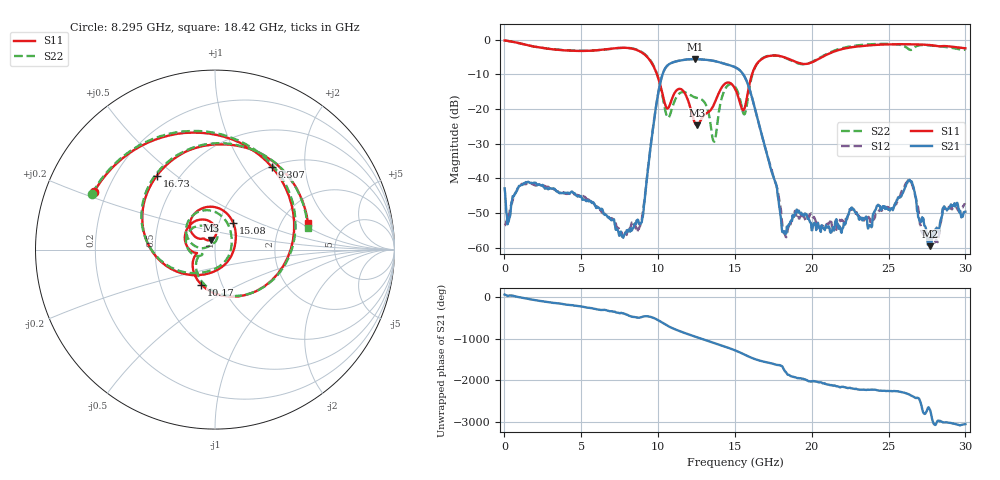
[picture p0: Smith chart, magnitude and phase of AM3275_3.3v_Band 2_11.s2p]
!Keysight Technologies,N5245B,MY58422270,A.16.20.02
!Date: Thursday, March 27, 2025 01:54:47
!Correction: S11(C  2-Port  )
!S21(C  2-Port  )
!S12(C  2-Port  )
!S22(C  2-Port  )
!S2P File: Measurements: S11, S21, S12, S22:
# Hz S  dB  R 50
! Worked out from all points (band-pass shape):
!   801 points, 10 MHz to 30 GHz, reference 50 ohm
!   highest |S21| = -5.59 dB at 12.38 GHz (marker M1); lowest = -59.6 dB at 27.71 GHz (marker M2)
!   |S21| within 3 dB of the highest: 10.42 GHz to 15.26 GHz (4.837 GHz wide, 37.7 % of centre)
!   lowest |S11| = -24.6 dB at 12.53 GHz (marker M3), VSWR 1.12, Z = 47.5 + j5.16 ohm
!   |S11| at or under -10 dB: 9.927 GHz to 16.11 GHz (6.183 GHz wide, 47.5 % of centre)
!   |S22| runs from -29.4 to -0.2 dB; largest |S21 - S12| = 0.0088
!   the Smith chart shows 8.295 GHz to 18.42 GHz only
!   S11 on the Smith chart (normalised r, x): 8.295 GHz: 0.15, +0.22; 9.307 GHz: 1.01, +1.36; 10.17 GHz: 0.80, -0.33; 15.08 GHz: 1.16, +0.36; 16.73 GHz: 0.38, +0.43; 18.42 GHz: 2.78, +1.17
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1e7  -0.20 -5.3  -42.87 49.9  -53.58 -84.8  -0.20 -6.2
9.097e8  -0.92 -86.4  -42.54 -10.0  -42.63 -6.4  -0.96 -86.3
2.071812e9  -2.08 -170.8  -41.58 -87.7  -42.06 -87.3  -2.08 -170.5
5.033325e9  -3.23 26.2  -45.60 123.8  -44.97 118.4  -3.18 25.1
6.832725e9  -2.63 -91.7  -51.58 12.4  -51.35 19.2  -2.68 -92.4
8.294738e9  -2.54 154.6  -55.01 -115.7  -52.72 -117.3  -2.48 155.5
9.3069e9  -5.05 55.6  -38.67 -107.2  -38.55 -105.5  -4.88 56.2
1.001916e10  -11.22 -72.6  -15.16 155.1  -15.13 154.9  -11.10 -68.5
1.016911e10  -13.54 -111.0  -11.92 122.0  -11.89 121.8  -13.69 -105.3
1.136871e10  -14.18 137.1  -6.04 -97.9  -6.03 -98.0  -15.55 165.9
1.238088e10  -23.88 96.9  -5.59 129.7  -5.58 129.7  -16.59 116.1
1.253082e10  -24.65 112.6  -5.60 111.2  -5.59 111.2  -16.78 112.7
1.346801e10  -20.01 143.2  -5.98 -2.3  -5.97 -2.5  -26.18 83.0
1.5005e10  -14.13 63.8  -7.92 159.1  -7.90 159.0  -13.54 90.2
1.507998e10  -14.85 56.1  -8.08 147.8  -8.06 147.8  -14.05 83.1
1.672942e10  -5.62 128.2  -27.11 -97.3  -27.19 -97.5  -5.53 129.9
1.841636e10  -5.37 16.1  -54.40 -55.8  -55.48 -76.4  -5.51 13.3
2.002832e10  -6.48 -124.8  -55.01 136.9  -50.77 145.5  -6.37 -128.1
2.253999e10  -2.20 102.7  -48.84 -24.1  -48.80 -20.3  -1.90 104.1
2.501416e10  -1.35 38.5  -48.96 -93.3  -48.55 -98.0  -1.19 36.5
2.771326e10  -1.53 -29.3  -59.57 166.1  -56.75 -18.8  -1.64 -28.7
3e10  -2.46 -110.9  -49.63 -160.2  -47.62 -174.0  -2.90 -108.8
